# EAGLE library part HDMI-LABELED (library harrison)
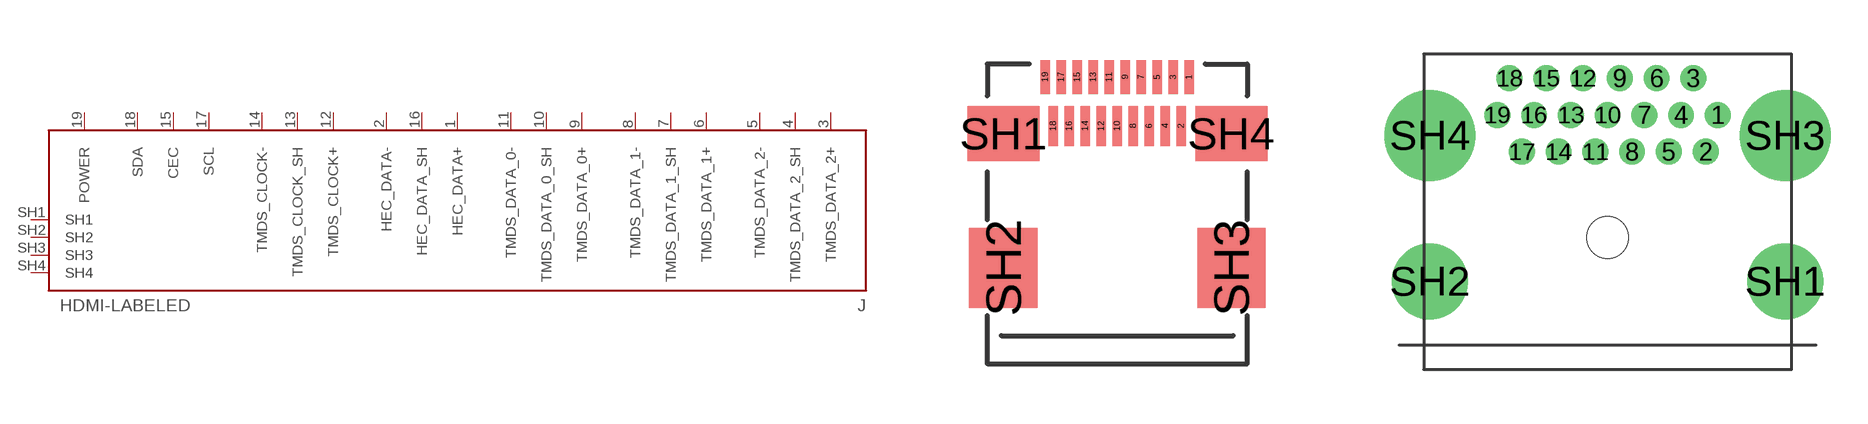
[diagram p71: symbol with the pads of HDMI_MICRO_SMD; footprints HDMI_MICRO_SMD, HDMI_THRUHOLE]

Designator prefix J

## HDMI-LABELED_D  [HDMI_MICRO_SMD]
1  HEC_DATA+
2  HEC_DATA-
3  TMDS_DATA_2+
4  TMDS_DATA_2_SH  pwr
5  TMDS_DATA_2-
6  TMDS_DATA_1+
7  TMDS_DATA_1_SH  pwr
8  TMDS_DATA_1-
9  TMDS_DATA_0+
10  TMDS_DATA_0_SH  pwr
11  TMDS_DATA_0-
12  TMDS_CLOCK+
13  TMDS_CLOCK_SH  pwr
14  TMDS_CLOCK-
15  CEC
16  HEC_DATA_SH  pwr
17  SCL
18  SDA
19  POWER  pwr
SH1  SH1  pwr
SH2  SH2  pwr
SH3  SH3  pwr
SH4  SH4  pwr

## HDMI-LABELED_A_THRUHOLE  [HDMI_THRUHOLE]
1  TMDS_DATA_2+
2  TMDS_DATA_2_SH  pwr
3  TMDS_DATA_2-
4  TMDS_DATA_1+
5  TMDS_DATA_1_SH  pwr
6  TMDS_DATA_1-
7  TMDS_DATA_0+
8  TMDS_DATA_0_SH  pwr
9  TMDS_DATA_0-
10  TMDS_CLOCK+
11  TMDS_CLOCK_SH  pwr
12  TMDS_CLOCK-
13  CEC
14  HEC_DATA-
15  SCL
16  SDA
17  HEC_DATA_SH  pwr
18  POWER  pwr
19  HEC_DATA+
SH1  SH1  pwr
SH2  SH2  pwr
SH3  SH3  pwr
SH4  SH4  pwr

## HDMI-LABELED_A  [HDMI_A_SMD]
Pads as for HDMI_THRUHOLE

## Footprint HDMI_MICRO_SMD (pad centres in mm)
smd 0.23 x 0.85: 1 1.8,3.475; 3 1.4,3.475; 5 1,3.475; 7 0.6,3.475; 9 0.2,3.475; 11 -0.2,3.475; 13 -0.6,3.475; 15 -1,3.475; 17 -1.4,3.475; 19 -1.8,3.475
smd 0.23 x 1: 2 1.6,2.25; 4 1.2,2.25; 6 0.8,2.25; 8 0.4,2.25; 10 0,2.25; 12 -0.4,2.25; 14 -0.8,2.25; 16 -1.2,2.25; 18 -1.6,2.25
smd 1.8 x 1.38: SH1 -2.85,2.06; SH4 2.85,2.06
smd 1.7 x 2: SH2 -2.85,-1.3; SH3 2.85,-1.3

## Footprint HDMI_THRUHOLE (pad centres in mm)
drill 0.55 pad 0.965: 1 4.5,5; 2 4,3.5; 3 3.5,6.5; 4 3,5; 5 2.5,3.5; 6 2,6.5; 7 1.5,5; 8 1,3.5; 9 0.5,6.5; 10 0,5; 11 -0.5,3.5; 12 -1,6.5; 13 -1.5,5; 14 -2,3.5; 15 -2.5,6.5; 16 -3,5; 17 -3.5,3.5; 18 -4,6.5; 19 -4.5,5
drill 2.1: SH1 7.25,-1.8; SH2 -7.25,-1.8
drill 2.7: SH3 7.25,4.16; SH4 -7.25,4.16
hole 1.7 at 0,0

## Footprint HDMI_A_SMD (pad centres in mm)
smd 0.3 x 1.9: 1 4.75,5; 2 4.25,5; 3 3.75,5; 4 3.25,5; 5 2.75,5; 6 2.25,5; 7 1.75,5; 8 1.25,5; 9 0.75,5; 10 0.25,5; 11 -0.25,5; 12 -0.75,5; 13 -1.25,5; 14 -1.75,5; 15 -2.25,5; 16 -2.75,5; 17 -3.25,5; 18 -3.75,5; 19 -4.25,5
drill 1.3: SH1 7.85,-0.9; SH2 -7.85,-0.9; SH3 7.25,4; SH4 -7.25,4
